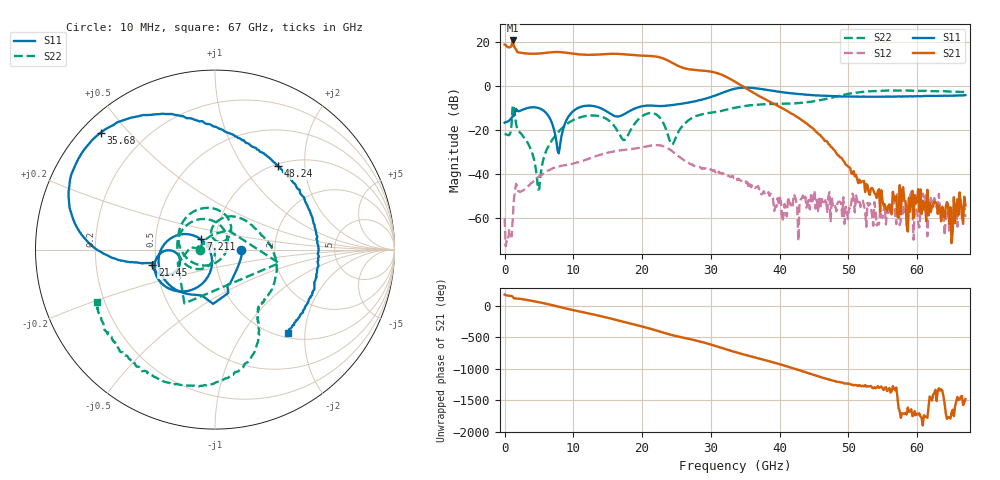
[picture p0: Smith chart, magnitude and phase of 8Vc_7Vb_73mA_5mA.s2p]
! MARKI MICROWAVE INC.
! Date:  05/05/2020
! Model Number:  APM-7099CH
! Description:  2-port Small Signal S-parameter data for APM-7099CH
! Frequency Range:  10 MHz to 67 GHz
! Port Configuration:  PORT 1: Input
!  PORT 2: Output
! Bias Condition: Vc = +8V, Vb = +7V
! APM-7099CH s2p files are only valid for small signal conditions (below -5 dBm input power)
!S2P File: Measurements: Mag<S11> Ang<S11>, Mag<S21> Ang<S21>, Mag<S12> Ang<S12>, Mag<S22> Ang<S22>!row 1
# Hz S  dB  R 50
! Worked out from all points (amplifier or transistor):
!   401 points, 10 MHz to 67 GHz, reference 50 ohm
!   highest |S21| = 20.6 dB at 1.182 GHz (marker M1)
!   |S21| within 3 dB of that: start of sweep to 474.2 MHz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
!   unconditionally stable (mu >= 1): start of sweep to end of sweep
!   at 11.06 GHz: K = 4.34, MAG = 14.9 dB, |S12| = -34.3 dB
!   at 33.51 GHz: K = 11.34, MAG = 8.4 dB, |S12| = -41.9 dB
!   at 67 GHz: K = 70259.77, MAG = -48.8 dB, |S12| = -59.4 dB
!   S11 on the Smith chart (normalised r, x): 10 MHz: 1.34, -0.01; 7.211 GHz: 0.85, +0.10; 21.45 GHz: 0.48, -0.09; 35.68 GHz: 0.05, +0.42; 48.24 GHz: 1.03, +1.46; 67 GHz: 1.08, -1.64
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1e7  -16.67 -1.5  18.71 178.4  -59.98 -45.5  -21.81 -176.9
1.182325e9  -13.72 -65.8  20.59 146.1  -60.82 76.1  -8.76 -11.9
1.68475e9  -10.39 -91.9  16.41 113.1  -44.34 -80.3  -17.30 174.8
4.6993e9  -9.83 -167.2  14.60 63.1  -41.80 -170.7  -41.19 138.4
7.211425e9  -20.01 143.8  15.34 3.0  -37.10 129.2  -23.20 -102.8
9.221125e9  -14.24 -109.3  14.94 -50.3  -35.65 85.9  -16.89 -130.5
1.123082e10  -9.34 -141.8  14.19 -98.5  -34.06 50.6  -14.01 -167.6
1.458032e10  -11.05 -178.5  14.43 -178.8  -30.60 -16.4  -14.52 115.2
1.592012e10  -13.56 -172.8  14.55 144.7  -29.59 -47.1  -18.05 68.4
1.74274e10  -12.74 -153.0  14.31 102.5  -28.96 -82.6  -24.54 -42.7
1.977205e10  -9.38 -156.8  13.74 37.9  -27.92 -136.9  -14.28 177.8
2.14468e10  -8.92 -166.4  13.51 -11.6  -26.95 177.6  -12.30 112.7
2.245165e10  -9.11 -168.5  13.03 -44.4  -26.86 145.1  -13.92 73.0
2.446135e10  -8.63 -168.3  10.33 -107.9  -29.77 80.7  -26.32 81.4
2.663852e10  -7.59 -169.6  7.64 -160.4  -34.69 39.5  -15.83 84.1
3.01555e10  -4.83 -175.4  6.38 99.7  -38.18 -10.7  -12.05 29.7
3.3505e10  -1.24 160.2  1.91 -12.8  -41.95 -65.1  -9.88 0.4
3.568218e10  -0.81 134.4  -2.21 -78.4  -44.58 -99.4  -8.76 -18.9
4.472582e10  -4.16 72.6  -18.96 -7.4  -52.30 -2.7  -7.08 -57.6
4.82428e10  -4.68 53.0  -30.53 -123.9  -56.84 -59.9  -4.78 -66.1
5.594665e10  -4.83 7.6  -53.75 137.7  -53.07 -153.1  -2.10 -108.6
6.7e10  -4.17 -48.9  -54.07 -40.4  -59.39 110.1  -2.87 -156.0
